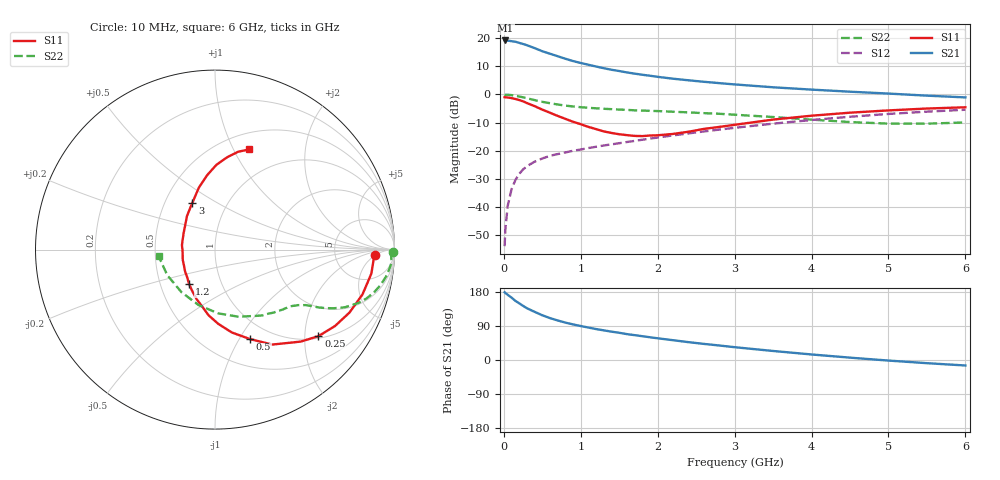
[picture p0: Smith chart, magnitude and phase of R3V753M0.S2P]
! SIEMENS Small Signal Semiconductors
! BFR181
! Si NPN RF Bipolar Junction Transistor in SOT23
! VCE = 0.75 V  IC = 3 mA
! Common Emitter S-Parameters:  May  1996
# GHz  S  MA  R  50
!  f  S11  S21  S12  S22
! GHz  MAG  ANG  MAG  ANG  MAG  ANG  MAG  ANG
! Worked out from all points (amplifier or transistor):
!   36 points, 10 MHz to 6 GHz, reference 50 ohm
!   highest |S21| = 19.2 dB at 20 MHz (marker M1)
!   |S21| within 3 dB of that: start of sweep to 425.4 MHz
!   unconditionally stable (mu >= 1): 1.208 GHz to 3.542 GHz
!   at 250 MHz: K = 0.32, MSG = 22.3 dB, |S12| = -26.7 dB
!   at 1.4 GHz: K = 1.06, MAG = 11.8 dB, |S12| = -17.8 dB
!   at 6 GHz: K = 0.91, MSG = 2.2 dB, |S12| = -5.5 dB
!   S11 on the Smith chart (normalised r, x): 10 MHz: 16, -4; 250 MHz: 1.06, -2.34; 500 MHz: 0.80, -1.11; 1.2 GHz: 0.70, -0.29; 3 GHz: 0.69, +0.39; 6 GHz: 0.68, +1.16
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0.01  0.8903 -1.8  9.004 178.7  0.002 91.1  0.9923 -0.8
0.02  0.8857 -3.4  9.096 176.7  0.004 90.3  0.9813 -1.7
0.05  0.8815 -8.7  9.049 172.1  0.0104 85.2  0.9862 -4.2
0.1  0.8588 -16.9  8.827 164.6  0.0205 81.0  0.9708 -8.1
0.15  0.8273 -25.1  8.643 156.1  0.03 74.9  0.9451 -11.9
0.25  0.7515 -39.9  7.87 142.9  0.0463 68.3  0.8865 -17.9
0.3  0.7008 -47.0  7.485 136.6  0.0527 65.9  0.8545 -20.3
0.4  0.6179 -58.9  6.653 127.1  0.0636 61.0  0.7907 -24.0
0.5  0.5356 -68.6  5.851 118.0  0.0725 58.3  0.7378 -26.3
0.6  0.4713 -78.5  5.283 110.6  0.0808 56.7  0.6963 -27.9
0.7  0.4141 -87.5  4.767 104.3  0.0868 55.4  0.6605 -29.2
0.8  0.367 -95.7  4.3 98.7  0.0928 54.5  0.6317 -30.0
0.9  0.3257 -102.5  3.913 93.9  0.0995 54.6  0.6096 -30.8
1.1  0.2639 -118.6  3.361 85.6  0.1112 54.6  0.5778 -32.4
1.2  0.241 -126.8  3.129 81.6  0.1172 54.7  0.5649 -33.2
1.6  0.1885 -162.2  2.455 68.3  0.1422 55.7  0.5297 -36.5
2.2  0.1981 151.8  1.9 52.2  0.1864 55.5  0.4909 -44.1
3  0.2877 116.2  1.504 33.8  0.2544 52.2  0.4349 -58.1
3.5  0.3563 104.7  1.337 23.8  0.3016 48.4  0.3958 -70.8
4.5  0.4728 89.0  1.116 6.2  0.4001 38.2  0.3221 -106.6
5.5  0.5602 76.7  0.949 -8.4  0.4931 25.5  0.3016 -151.5
6  0.5898 71.1  0.884 -14.5  0.5334 18.4  0.3166 -173.4
